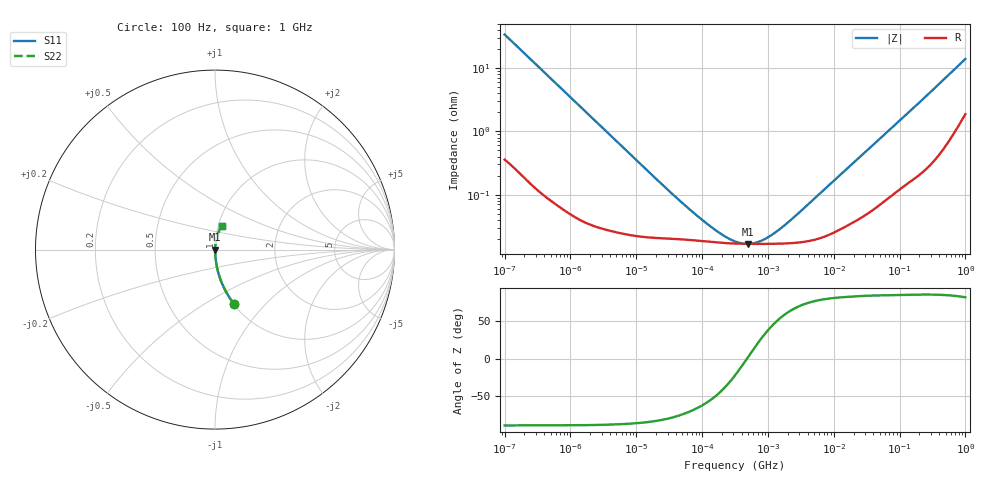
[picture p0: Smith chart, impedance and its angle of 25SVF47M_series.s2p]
!  *** S-Parameter ***
!  Copyright (C) Panasonic Industry
!  Conductive Polymer Aluminum Soild Capacitor (OS-CON)
!  Parts No. 25SVF47M
!  Connection Mode : Series
!  1  o---||---o  2
!  GND o--------o GND
!  Conditions : Temperature = 20 degC  DC Bias = 0 V
! Frequency Range : 100Hz  -  1GHz  [ 401 Steps ]
# Hz S RI R 50
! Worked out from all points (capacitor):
!   401 points, 100 Hz to 1 GHz, reference 50 ohm
!   read as one part in series: C = 46.3 uF near 108.4 Hz
!   lowest |Z| = 16.6 mohm at 492.6 kHz (marker M1)
!   series resonance near 479.9 kHz, so ESL is about 2.4 nH
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100  0.1078 -0.3049  0.8922 0.3049  0.8922 0.3049  0.1078 -0.3049
108.3927  0.0936 -0.286  0.9064 0.286  0.9064 0.286  0.0936 -0.286
168.8496  0.0419 -0.195  0.9581 0.195  0.9581 0.195  0.0419 -0.195
321.7363  0.0125 -0.106  0.9875 0.106  0.9875 0.106  0.0125 -0.106
638.2635  0.00361 -0.0541  0.9964 0.0541  0.9964 0.0541  0.00361 -0.0541
1487.647  0.000932 -0.0234  0.9991 0.0234  0.9991 0.0234  0.000932 -0.0234
22130.95  0.000207 -0.0016  0.9998 0.0016  0.9998 0.0016  0.000207 -0.0016
53703.18  0.000195 -0.000663  0.9998 0.000663  0.9998 0.000663  0.000195 -0.000663
115478.2  0.000181 -0.000305  0.9998 0.000305  0.9998 0.000305  0.000181 -0.000305
203001.9  0.000172 -0.000154  0.9998 0.000154  0.9998 0.000154  0.000172 -0.000154
316227.8  0.000168 -6.9e-05  0.9998 6.9e-05  0.9998 6.9e-05  0.000168 -6.9e-05
402717  0.000167 -2.84e-05  0.9998 2.84e-05  0.9998 2.84e-05  0.000167 -2.84e-05
492606.3  0.000166 4.26e-06  0.9998 -4.26e-06  0.9998 -4.26e-06  0.000166 4.26e-06
602559.6  0.000166 3.72e-05  0.9998 -3.72e-05  0.9998 -3.72e-05  0.000166 3.72e-05
737055.2  0.000166 7.17e-05  0.9998 -7.17e-05  0.9998 -7.17e-05  0.000166 7.17e-05
1148154  0.000166 0.00016  0.9998 -0.00016  0.9998 -0.00016  0.000166 0.00016
2018366  0.000169 0.000321  0.9998 -0.000321  0.9998 -0.000321  0.000169 0.000321
4704354  0.000189 0.00078  0.9998 -0.00078  0.9998 -0.00078  0.000189 0.00078
6.99842e7  0.00102 0.0105  0.999 -0.0105  0.999 -0.0105  0.00102 0.0105
3.235937e8  0.00536 0.0455  0.9946 -0.0455  0.9946 -0.0455  0.00536 0.0455
8.51138e8  0.0273 0.1142  0.9727 -0.1142  0.9727 -0.1142  0.0273 0.1142
1e9  0.0364 0.1317  0.9636 -0.1317  0.9636 -0.1317  0.0364 0.1317
